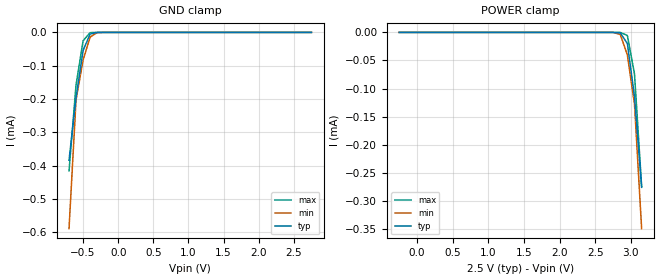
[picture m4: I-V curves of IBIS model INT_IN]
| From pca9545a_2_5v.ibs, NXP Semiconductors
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[Model]   INT_IN
Model_type Input
Vinh=2.1
Vinl=0.9
C_comp   1.73p   1.73p   1.73p
[Temperature Range] 27   85   -40
[Voltage Range]   2.5   2.25   2.75
[POWER Clamp Reference]2.5   2.25   2.75
[GND Clamp Reference]0   0   0
[GND Clamp]
-700mV    -384.1uA   -589.5uA   -416uA
-600mV    -196.2uA   -202.7uA   -157.7uA
-500mV    -54.35uA   -83.42uA   -25.32uA
-400mV    -5.044uA   -14.16uA   -762nA
-300mV    -137.5nA   -707nA     -7.814nA
-200mV    -2.331nA   -17.81nA   -62.01pA
2.75V     9.055pA    20.47pA    8.255pA
[POWER Clamp]
-250mV    9.055pA    20.47pA    8.255pA
2.75V     -18.34nA   -116.7nA   -704pA
2.85V     -926.5nA   -3.623uA   -82.04nA
2.95V     -19.81uA   -40.17uA   -5.446uA
3.05V     -114.3uA   -128uA     -74.05uA
3.15V     -275.8uA   -349.4uA   -273.9uA
